| IBIS file 71660dr.ibs created by s2ibis2 version 1.2
| North Carolina State University Electronics Research Laboratory  1995
[IBIS ver]   2.1
[File name]   71660dr.ibs
[File Rev]   1.2
[Date]   11/10/2004
[Source]   Integrated Device Technology, Inc.
[Notes]   1.Temperatures: typ=25C, min=100C, max=0C
   2.Ramp rates based on 50 ohm load.
   3.The model for the open-drain dta pin does not reflect a
   pulsed pull-up device which aides the output on highz.
[Disclaimer] Integrated Device Technology, Inc. ("IDT") hereby grants the
   user of this IBIS model a non-exclusive, nontransferable
   license to use this IBIS model under the following terms. The
   user is granted this license only to use the IBIS model and is
   not granted rights to sell, copy (except as needed to run the
   IBIS model), rent, lease or sub-license the IBIS model in
   whole or in part, or in modified form to anyone. The User may
   modify the IBIS model to suit its specific applications, but
   rights to derivative works and such modifications shall belong
   to IDT. This IBIS model is provided on an AS IS" basis and IDT
   makes absolutely no warranty with respect to the information
   contained herein. IDT DISCLAIMS AND CUSTOMER WAIVES ALL
   WARRANTIES, EXPRESS AND IMPLIED, INCLUDING WARRANTIES OF
   MERCHANTABILITY AND FITNESS FOR A PARTICULAR PURPOSE. THE
   ENTIRE RISK AS TO QUALITY AND PERFORMANCE IS WITH THE USER
   ACCORDINGLY, IN NO EVENT SHALL IDT BE LIABLE FOR ANY DIRECT OR
   INDIRECT DAMAGES, WHETHER IN CONTRACT OR TORT, INCLUDING ANY
   LOST PROFITS OR OTHER INCIDENTAL, CONSEQUENTIAL, EXEMPLARY, OR
   PUNITIVE DAMAGES ARISING OUT OF THE USE OR APPLICATION OF THE
   IBIS model. Further, IDT reserves the right to make changes
   without notice to any product herein to improve reliability,
   function, or design. IDT does not convey any license under
   patent rights or any other intellectual property rights,
   including those of third parties. IDT is not obligated to
   provide maintenance or support for the licensed IBIS model.
[Copyright]   Copyright 2001, Integrated Device Technology, Inc. all rights
   reserved
|   Component 72v71660
[Component]   72v71660
[Manufacturer]   Integrated Device Technology
[Package]
| DR208
| variable   typ   min   max
R_pkg   129.8m   50.0m   0.30
L_pkg   9.76nH   9.0nH   14.0nH
C_pkg   1.234pF   0.74pF   1.3pF
[Pin]   signal_name   model_name   R_pin   L_pin   C_pin
207   ode   inpad1
208   resetx   inpad1
2   clk   inpad1
3   foi   inpad1
4   fe_hclk   inpad1
5   wfps   inpad1
6   tms   inpad2
7   tdi   inpad2
8   tdo   iopad1
9   tck   inpad1
10   trstx   inpad2
11   dsx   inpad1
12   csx   inpad1
13   rwx   inpad1
15   a0   inpad1
16   a1   inpad1
17   a2   inpad1
18   a3   inpad1
19   a4   inpad1
20   a5   inpad1
21   a6   inpad1
22   a7   inpad1
23   a8   inpad1
24   a9   inpad1
25   a10   inpad1
26   a11   inpad1
27   a12   inpad1
28   a13   inpad1
29   a14   inpad1
30   a15   inpad1
32   dtax   outpad3
33   d15   iopad2
34   d14   iopad2
35   d13   iopad2
36   d12   iopad2
39   d11   iopad2
40   d10   iopad2
41   d9   iopad2
44   d8   iopad2
45   d7   iopad2
46   d6   iopad2
47   d5   iopad2
48   d4   iopad2
51   d3   iopad2
52   d2   iopad2
53   d1   iopad2
54   d0   iopad2
55   rx63   inpad1
56   rx62   inpad1
57   rx61   inpad1
58   rx60   inpad1
59   rx59   inpad1
60   rx58   inpad1
61   rx57   inpad1
62   rx56   inpad1
63   tx63   iopad1
64   tx62   iopad1
65   tx61   iopad1
66   tx60   iopad1
69   tx59   iopad1
70   tx58   iopad1
71   tx57   iopad1
72   tx56   iopad1
75   tx55   iopad1
76   tx54   iopad1
77   tx53   iopad1
78   tx52   iopad1
81   tx51   iopad1
82   tx50   iopad1
83   tx49   iopad1
84   tx48   iopad1
85   rx55   inpad1
86   rx54   inpad1
87   rx53   inpad1
88   rx52   inpad1
89   rx51   inpad1
90   rx50   inpad1
91   rx49   inpad1
92   rx48   inpad1
93   rx47   inpad1
94   rx46   inpad1
95   rx45   inpad1
96   rx44   inpad1
97   rx43   inpad1
98   rx42   inpad1
99   rx41   inpad1
100   rx40   inpad1
101   tx47   iopad1
102   tx46   iopad1
103   tx45   iopad1
104   tx44   iopad1
107   tx43   iopad1
108   tx42   iopad1
109   tx41   iopad1
110   tx40   iopad1
113   tx39   iopad1
114   tx38   iopad1
115   tx37   iopad1
116   tx36   iopad1
119   tx35   iopad1
120   tx34   iopad1
121   tx33   iopad1
122   tx32   iopad1
123   rx39   inpad1
124   rx38   inpad1
125   rx37   inpad1
126   rx36   inpad1
127   rx35   inpad1
128   rx34   inpad1
129   rx33   inpad1
130   rx32   inpad1
131   rx31   inpad1
132   rx30   inpad1
133   rx29   inpad1
134   rx28   inpad1
135   rx27   inpad1
136   rx26   inpad1
137   rx25   inpad1
138   rx24   inpad1
139   tx31   iopad1
140   tx30   iopad1
141   tx29   iopad1
142   tx28   iopad1
145   tx27   iopad1
146   tx26   iopad1
147   tx25   iopad1
148   tx24   iopad1
151   tx23   iopad1
152   tx22   iopad1
153   tx21   iopad1
154   tx20   iopad1
157   tx19   iopad1
158   tx18   iopad1
159   tx17   iopad1
160   tx16   iopad1
161   rx23   inpad1
162   rx22   inpad1
163   rx21   inpad1
164   rx20   inpad1
165   rx19   inpad1
166   rx18   inpad1
167   rx17   inpad1
168   rx16   inpad1
169   rx15   inpad1
170   rx14   inpad1
171   rx13   inpad1
172   rx12   inpad1
173   rx11   inpad1
174   rx10   inpad1
175   rx9   inpad1
176   rx8   inpad1
177   tx15   iopad1
178   tx14   iopad1
179   tx13   iopad1
180   tx12   iopad1
183   tx11   iopad1
184   tx10   iopad1
185   tx9   iopad1
186   tx8   iopad1
189   tx7   iopad1
190   tx6   iopad1
191   tx5   iopad1
192   tx4   iopad1
195   tx3   iopad1
196   tx2   iopad1
197   tx1   iopad1
198   tx0   iopad1
199   rx7   inpad1
200   rx6   inpad1
201   rx5   inpad1
202   rx4   inpad1
203   rx3   inpad1
204   rx2   inpad1
205   rx1   inpad1
206   rx0   inpad1
194   vdd   POWER
188   vdd   POWER
182   vdd   POWER
156   vdd   POWER
150   vdd   POWER
144   vdd   POWER
117   vdd   POWER
111   vdd   POWER
105   vdd   POWER
79   vdd   POWER
73   vdd   POWER
67   vdd   POWER
49   vdd   POWER
42   vdd   POWER
37   vdd   POWER
14   vdd   POWER
193   vss   GND
187   vss   GND
181   vss   GND
155   vss   GND
149   vss   GND
143   vss   GND
118   vss   GND
112   vss   GND
106   vss   GND
80   vss   GND
74   vss   GND
68   vss   GND
50   vss   GND
43   vss   GND
38   vss   GND
1   vss   GND
| in   in   dummy_model
| oe   oe   dummy_model
[Pin Mapping]  pulldown_ref   pullup_ref   gnd_clamp_ref   power_clamp_ref
207   vss   vdd
208   vss   vdd
2   vss   vdd
3   vss   vdd
4   vss   vdd
5   vss   vdd
6   vss   vdd
7   vss   vdd
8   vss   vdd
9   vss   vdd
10   vss   vdd
11   vss   vdd
12   vss   vdd
13   vss   vdd
15   vss   vdd
16   vss   vdd
17   vss   vdd
18   vss   vdd
19   vss   vdd
20   vss   vdd
21   vss   vdd
22   vss   vdd
23   vss   vdd
24   vss   vdd
25   vss   vdd
26   vss   vdd
27   vss   vdd
28   vss   vdd
29   vss   vdd
30   vss   vdd
32   vss   vdd
33   vss   vdd
34   vss   vdd
35   vss   vdd
36   vss   vdd
39   vss   vdd
40   vss   vdd
41   vss   vdd
44   vss   vdd
45   vss   vdd
46   vss   vdd
47   vss   vdd
48   vss   vdd
51   vss   vdd
52   vss   vdd
53   vss   vdd
54   vss   vdd
55   vss   vdd
56   vss   vdd
57   vss   vdd
58   vss   vdd
59   vss   vdd
60   vss   vdd
61   vss   vdd
62   vss   vdd
63   vss   vdd
64   vss   vdd
65   vss   vdd
66   vss   vdd
69   vss   vdd
70   vss   vdd
71   vss   vdd
72   vss   vdd
75   vss   vdd
76   vss   vdd
77   vss   vdd
78   vss   vdd
81   vss   vdd
82   vss   vdd
83   vss   vdd
84   vss   vdd
85   vss   vdd
86   vss   vdd
87   vss   vdd
88   vss   vdd
89   vss   vdd
90   vss   vdd
91   vss   vdd
92   vss   vdd
93   vss   vdd
94   vss   vdd
95   vss   vdd
96   vss   vdd
97   vss   vdd
98   vss   vdd
99   vss   vdd
100   vss   vdd
101   vss   vdd
102   vss   vdd
103   vss   vdd
104   vss   vdd
107   vss   vdd
108   vss   vdd
109   vss   vdd
110   vss   vdd
113   vss   vdd
114   vss   vdd
115   vss   vdd
116   vss   vdd
119   vss   vdd
120   vss   vdd
121   vss   vdd
122   vss   vdd
123   vss   vdd
124   vss   vdd
125   vss   vdd
126   vss   vdd
127   vss   vdd
128   vss   vdd
129   vss   vdd
130   vss   vdd
131   vss   vdd
132   vss   vdd
133   vss   vdd
134   vss   vdd
135   vss   vdd
136   vss   vdd
137   vss   vdd
138   vss   vdd
139   vss   vdd
140   vss   vdd
141   vss   vdd
142   vss   vdd
145   vss   vdd
146   vss   vdd
147   vss   vdd
148   vss   vdd
151   vss   vdd
152   vss   vdd
153   vss   vdd
154   vss   vdd
157   vss   vdd
158   vss   vdd
159   vss   vdd
160   vss   vdd
161   vss   vdd
162   vss   vdd
163   vss   vdd
164   vss   vdd
165   vss   vdd
166   vss   vdd
167   vss   vdd
168   vss   vdd
169   vss   vdd
170   vss   vdd
171   vss   vdd
172   vss   vdd
173   vss   vdd
174   vss   vdd
175   vss   vdd
176   vss   vdd
177   vss   vdd
178   vss   vdd
179   vss   vdd
180   vss   vdd
183   vss   vdd
184   vss   vdd
185   vss   vdd
186   vss   vdd
189   vss   vdd
190   vss   vdd
191   vss   vdd
192   vss   vdd
195   vss   vdd
196   vss   vdd
197   vss   vdd
198   vss   vdd
199   vss   vdd
200   vss   vdd
201   vss   vdd
202   vss   vdd
203   vss   vdd
204   vss   vdd
205   vss   vdd
206   vss   vdd
194   nc   vdd
188   nc   vdd
182   nc   vdd
156   nc   vdd
150   nc   vdd
144   nc   vdd
117   nc   vdd
111   nc   vdd
105   nc   vdd
79   nc   vdd
73   nc   vdd
67   nc   vdd
49   nc   vdd
42   nc   vdd
37   nc   vdd
14   nc   vdd
193   vss   nc
187   vss   nc
181   vss   nc
155   vss   nc
149   vss   nc
143   vss   nc
118   vss   nc
112   vss   nc
106   vss   nc
80   vss   nc
74   vss   nc
68   vss   nc
50   vss   nc
43   vss   nc
38   vss   nc
1   vss   nc
| Models and submodels in the file (5): inpad1 (Input), inpad2 (Input), iopad1 (3-state), iopad2 (3-state), outpad3 (Open_drain)
